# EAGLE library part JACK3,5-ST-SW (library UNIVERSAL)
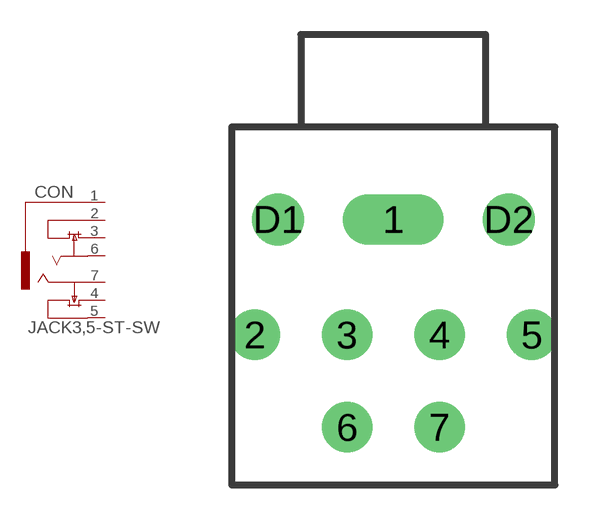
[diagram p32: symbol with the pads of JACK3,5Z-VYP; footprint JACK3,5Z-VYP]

Designator prefix CON

## JACK3,5-ST-SW  [JACK3,5Z-VYP]
1  1  pas
2  2  pas
3  3  pas
4  4  pas
5  5  pas
6  6  pas
7  7  pas

## Footprint JACK3,5Z-VYP (pad centres in mm)
drill 0.8 pad 2.184 long: 1 6,5
drill 0.8 pad 2.184: 2 0,0; 3 4,0; 4 8,0; 5 12,0; 6 4,-4; 7 8,-4
drill 1.5 pad 2.184: D1 1,5; D2 11,5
